FUNCTION_BLOCK Example01_longaxismotion //2x1 flyways w/ 1 xbots - linear, arc target, block buffer, release buffer, clear macro, save macro, run macro
VAR_INPUT
	Execute : BOOL;
END_VAR
VAR_OUTPUT
	Done : BOOL;
END_VAR
VAR_IN_OUT
	PM_Controller : PMControllerType;	// the planar motor controller to use
END_VAR
VAR
	PMC_XYMotion1: PMC_XYMotion;
	PMC_ArcMotionTarget1 : PMC_ArcMotionTarget;
	PMC_XYMotion2 : PMC_XYMotion;
	PMC_ArcMotionTarget2 : PMC_ArcMotionTarget;
	PMC_XYMotion3 : PMC_XYMotion;
	PMC_MotionBufferCtrl1 : PMC_MotionBufferCtrl;
	PMC_ArcMotionTarget3 : PMC_ArcMotionTarget;
	PMC_XYMotion4 : PMC_XYMotion;
	PMC_ArcMotionTarget4 : PMC_ArcMotionTarget;
	PMC_XYMotion5 : PMC_XYMotion;
	PMC_MotionBufferCtrl2 : PMC_MotionBufferCtrl;
	PMC_ClearMacro1 : PMC_ClearMacro;
	PMC_ArcMotionTarget5 : PMC_ArcMotionTarget;
	PMC_XYMotion6 : PMC_XYMotion;
	PMC_ArcMotionTarget6 : PMC_ArcMotionTarget;
	PMC_XYMotion7 : PMC_XYMotion;
	PMC_SaveMacro1 : PMC_SaveMacro;
	PMC_RunMacro1 : PMC_RunMacro;
END_VAR

//2x1 flyways w/ 1 xbots - linear, arc target, block buffer, release buffer, clear macro, save macro, run macro

//move xbot 1 to 120,180
PMC_XYMotion1(Execute := Execute,cmdLB := 1,XbotID := 1,Mode := 0,Type_ := 0,PosX := 0.12,PosY := 0.18,EndVel := 0,MaxVel := 1.0,MaxAcc := 10,PM_Controller := PM_Controller);

//arc motion counter clockwise to 120,60
PMC_ArcMotionTarget1(Execute := PMC_XYMotion1.Done,cmdLB := 2,XbotID := 1,Mode := 0,AType := 0,Dir := 1,EndVel := 0,MaxVel := 1,MaxAcc := 10,PosX := 0.12,PosY := 0.06,Radius := 0.06,PM_Controller := PM_Controller);

//linear motion to 360,60
PMC_XYMotion2(Execute := PMC_ArcMotionTarget1.Done,cmdLB := 3,XbotID := 1,Mode := 0,Type_ := 0,PosX := 0.36,PosY := 0.06,EndVel := 0,MaxVel := 1,MaxAcc := 10,PM_Controller := PM_Controller);

//arc motion to 360,180
PMC_ArcMotionTarget2(Execute := PMC_XYMotion2.Done,cmdLB := 4,XbotID := 1,Mode := 0,AType := 0,Dir := 1,EndVel := 0,MaxVel := 1.0,MaxAcc := 10,PosX := 0.36,PosY := 0.18,Radius := 0.06,PM_Controller := PM_Controller);

//linear motion to 120,180
PMC_XYMotion3(Execute := PMC_ArcMotionTarget2.Done,cmdLB := 5,XbotID := 1,Mode := 0,Type_ := 0,PosX := 0.12,PosY := 0.18,EndVel := 0,MaxVel := 1,MaxAcc := 10,PM_Controller := PM_Controller);

//block xbot 1 motion buffer	
PMC_MotionBufferCtrl1(Execute := PMC_XYMotion3.Done,Level := 0,XbotID := 1,PM_Controller := PM_Controller);

//arc motion to 120,60 non-zero ending speed
PMC_ArcMotionTarget3(Execute := PMC_MotionBufferCtrl1.Done,cmdLB := 7,XbotID := 1,Mode := 0,AType := 0,Dir := 1,EndVel := 1,MaxVel := 1,MaxAcc := 10,PosX := 0.12,PosY := 0.06,Radius := 0.06,PM_Controller := PM_Controller);

//linear motion to 360,60 non-zero ending speed
PMC_XYMotion4(Execute := PMC_ArcMotionTarget3.Ack,cmdLB := 8,XbotID := 1,Mode := 0,Type_ := 0,PosX := 0.36,PosY := 0.06,EndVel := 1,MaxVel := 1,MaxAcc := 10,PM_Controller := PM_Controller);

//arc motion to 360,180 non-zero ending speed
PMC_ArcMotionTarget4(Execute := PMC_XYMotion4.Ack,cmdLB := 9,XbotID := 1,Mode := 0,AType := 0,Dir := 1,EndVel := 1,MaxVel := 1,MaxAcc := 10,PosX := 0.36,PosY := 0.18,Radius := 0.06,PM_Controller := PM_Controller);

//linear move to 120,180 zero ending speed
PMC_XYMotion5(Execute := PMC_ArcMotionTarget4.Ack,cmdLB := 10,XbotID := 1,Mode := 0,Type_ := 0,PosX := 0.12,PosY := 0.18,EndVel := 0,MaxVel := 1,MaxAcc := 10,PM_Controller := PM_Controller);

//unblock xbot 1 buffer
PMC_MotionBufferCtrl2(Execute := PMC_XYMotion5.Ack,Level := 1,XbotID := 1,PM_Controller := PM_Controller);

//clear macro 128
PMC_ClearMacro1(Execute := PMC_MotionBufferCtrl2.Done,MacroID := 128,PM_Controller := PM_Controller);

//arc motion to 120,60 non-zero ending speed (macro 128)
PMC_ArcMotionTarget5(Execute := PMC_ClearMacro1.Done,cmdLB := 13,XbotID := 128,Mode := 0,AType := 0,Dir := 1,EndVel := 1,MaxVel := 1,MaxAcc := 10,PosX := 0.12,PosY := 0.06,Radius := 0.06,PM_Controller := PM_Controller);

//linear motion to 360,60 non-zero ending speed (macro 128)
PMC_XYMotion6(Execute := PMC_ArcMotionTarget5.Done,cmdLB := 14,XbotID := 128,Mode := 0,Type_ := 0,PosX := 0.36,PosY := 0.06,EndVel := 1,MaxVel := 1,MaxAcc := 10,PM_Controller := PM_Controller);

//arc motion to 360,180 non-zero ending speed (macro 128)
PMC_ArcMotionTarget6(Execute := PMC_XYMotion6.Done,cmdLB := 15,XbotID := 128,Mode := 0,AType := 0,Dir := 1,EndVel := 1,MaxVel := 1,MaxAcc := 10,PosX := 0.36,PosY := 0.18,Radius := 0.06,PM_Controller := PM_Controller);

//linear move to 120,180 zero ending speed
PMC_XYMotion7(Execute := PMC_ArcMotionTarget6.Done,cmdLB := 16,XbotID := 128,Mode := 0,Type_ := 0,PosX := 0.12,PosY := 0.18,EndVel := 0,MaxVel := 1,MaxAcc := 10,PM_Controller := PM_Controller);

//save macro 128
PMC_SaveMacro1(Execute := PMC_XYMotion7.Done,MacroID := 128,PM_Controller := PM_Controller);

//run macro 128 using xbot 1
PMC_RunMacro1(Execute := PMC_SaveMacro1.Done AND PMC_XYMotion5.Done,cmdLB := 18,MacroID := 128,XbotID := 1,PM_Controller := PM_Controller);


Done := PMC_RunMacro1.Done;

END_FUNCTION_BLOCK
